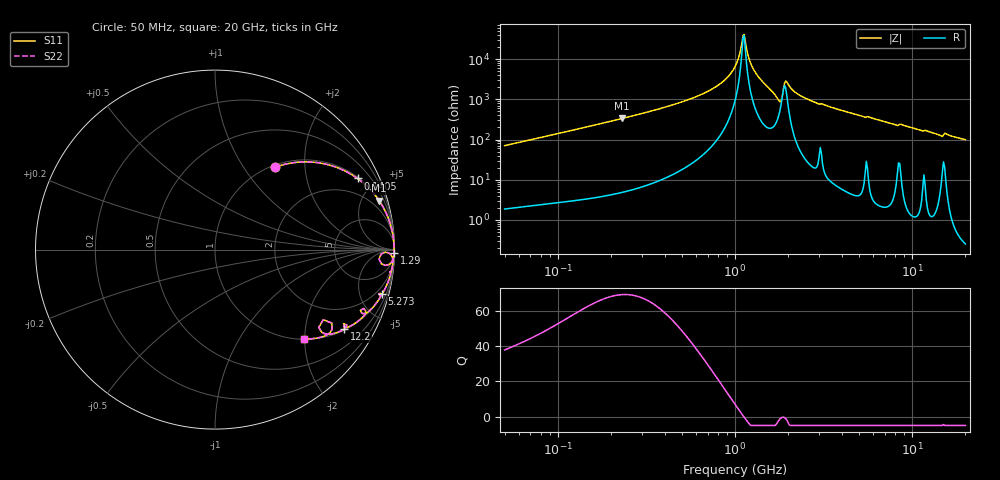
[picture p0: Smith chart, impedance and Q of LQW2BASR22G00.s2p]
!Murata Part Number: LQW2BASR22G00
!These Parameters are Measured in Series Mode Connection
!  o--[Z]--o
!Port1  Port2
!  o-------o
!Freq. Start=50[MHz] Stop=20[GHz], 401[Steps]
# Hz S RI R 50
!Freq.(Hz) S11(Real) S11(Imag) S21(Real) S21(Imag) S12(Real) S12(Imag) S22(Real) S22(Imag)
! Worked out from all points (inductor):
!   401 points, 50 MHz to 20 GHz, reference 50 ohm
!   read as one part in series: L = 223 nH near 51.52 MHz
!   highest Q = 69.2 at 230.4 MHz (marker M1), where L = 231 nH
!   self-resonance near 1.111 GHz
!   S11 on the Smith chart (normalised r, x): 50 MHz: 1.04, +1.41; 140.5 MHz: 1.06, +3.98; 1.29 GHz: open; 5.273 GHz: 1.11, -7.52; 12.2 GHz: 1.04, -3.24; 20 GHz: 1.01, -1.98
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5e7  0.3358 0.4592  0.6642 -0.4592  0.6642 -0.4592  0.3358 0.4592
1.364002e8  0.7842 0.4032  0.2158 -0.4032  0.2158 -0.4032  0.7842 0.4032
1.405482e8  0.7943 0.3962  0.2057 -0.3962  0.2057 -0.3962  0.7943 0.3962
2.304068e8  0.9145 0.2725  0.0855 -0.2725  0.0855 -0.2725  0.9145 0.2725
3.721004e8  0.9685 0.1668  0.0315 -0.1668  0.0315 -0.1668  0.9685 0.1668
7.30116e8  0.9946 0.0572  0.00543 -0.0572  0.00543 -0.0572  0.9946 0.0572
8.870719e8  0.9969 0.0309  0.00308 -0.0309  0.00308 -0.0309  0.9969 0.0309
1e9  0.9976 0.0151  0.00239 -0.0151  0.00239 -0.0151  0.9976 0.0151
1.045961e9  0.9977 0.00917  0.00227 -0.00917  0.00227 -0.00917  0.9977 0.00917
1.094034e9  0.9978 0.00318  0.00224 -0.00318  0.00224 -0.00318  0.9978 0.00318
1.127304e9  0.9977 -0.000842  0.00227 0.000842  0.00227 0.000842  0.9977 -0.000842
1.214974e9  0.9975 -0.0111  0.00253 0.0111  0.00253 0.0111  0.9975 -0.0111
1.289994e9  0.997 -0.0196  0.00299 0.0196  0.00299 0.0196  0.997 -0.0196
1.766834e9  0.9483 -0.0875  0.0517 0.0875  0.0517 0.0875  0.9483 -0.0875
1.820564e9  0.9139 -0.0532  0.0861 0.0532  0.0861 0.0532  0.9139 -0.0532
1.962148e9  0.9826 -0.0319  0.0174 0.0319  0.0174 0.0319  0.9826 -0.0319
2.211938e9  0.9911 -0.0682  0.00893 0.0682  0.00893 0.0682  0.9911 -0.0682
2.728004e9  0.9854 -0.1088  0.0146 0.1088  0.0146 0.1088  0.9854 -0.1088
5.273168e9  0.9306 -0.2466  0.0694 0.2466  0.0694 0.2466  0.9306 -0.2466
7.442007e9  0.8697 -0.3323  0.1303 0.3323  0.1303 0.3323  0.8697 -0.3323
1.220001e10  0.7212 -0.4423  0.2788 0.4423  0.2788 0.4423  0.7212 -0.4423
2e10  0.4954 -0.4987  0.5046 0.4987  0.5046 0.4987  0.4954 -0.4987
